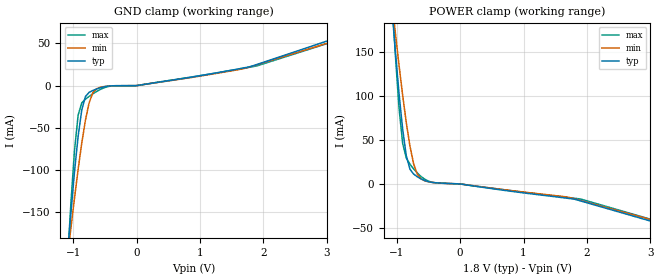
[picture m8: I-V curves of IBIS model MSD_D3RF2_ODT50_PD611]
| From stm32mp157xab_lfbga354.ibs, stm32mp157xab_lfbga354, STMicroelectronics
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[Model] MSD_D3RF2_ODT50_PD611
Model_type   Input
C_comp 2.328pF   2.289pF   2.357pF
Vinh = 1.150V
Vinl = 650.000mV
[Temperature Range]   25.000   125.000   -40.000
[Voltage Range]   1.800V   1.700V   1.900V
[GND Clamp Reference]   0.00V   0.00V   0.00V
[POWER Clamp Reference]   1.800V   1.700V   1.900V
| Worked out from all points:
|   GND clamp passes 1 mA (typ) near -0.48 V on its own axis
|   POWER clamp passes 1 mA (typ) near -0.31 V on its own axis
[GND Clamp]
-1.785V   -920.1mA   -680.6mA   -1.291A
-1.094V   -205.2mA   -206.6mA   -215.4mA
-1.036V   -151.5mA   -169.3mA   -140.1mA
-978.8mV  -102.2mA   -133.3mA   -77.09mA
-921.2mV  -59.95mA   -99.04mA   -34.92mA
-863.6mV  -28.6mA    -67.76mA   -20.39mA
-806.1mV  -12.9mA    -40.87mA   -16.02mA
-748.5mV  -7.982mA   -20.51mA   -12.78mA
-690.9mV  -5.748mA   -8.604mA   -9.786mA
-575.8mV  -2.62mA    -2.02mA    -4.64mA
1.785V    22.38mA    22.16mA    21.76mA
3.57V     67.03mA    63.08mA    63.28mA
[Power Clamp]
-1.77V    921.7mA    689.6mA    1.288A
-1.079V   203mA      209.3mA    218mA
-1.021V   150.6mA    171.7mA    146.8mA
-963.6mV  103.1mA    135.2mA    86.48mA
-906.1mV  62.26mA    100.8mA    46.12mA
-848.5mV  31.85mA    69.47mA    29.37mA
-790.9mV  16.74mA    42.87mA    22.42mA
-733.3mV  11.22mA    22.97mA    17.08mA
-618.2mV  5.734mA    5.806mA    8.558mA
-387.9mV  1.358mA    1.28mA     1.188mA
1.8V      -17.31mA   -16.97mA   -16.28mA
3.585V    -54.39mA   -51.94mA   -52.35mA
